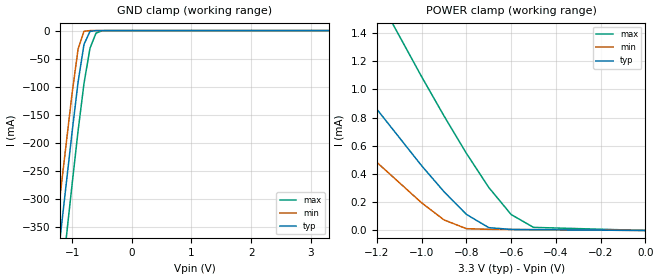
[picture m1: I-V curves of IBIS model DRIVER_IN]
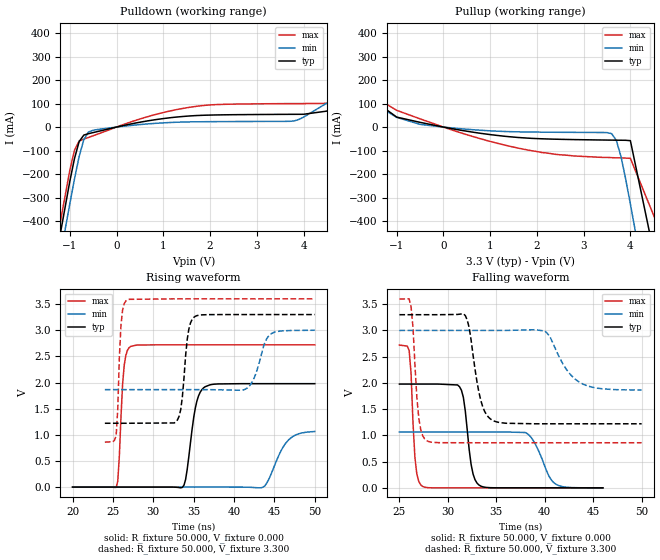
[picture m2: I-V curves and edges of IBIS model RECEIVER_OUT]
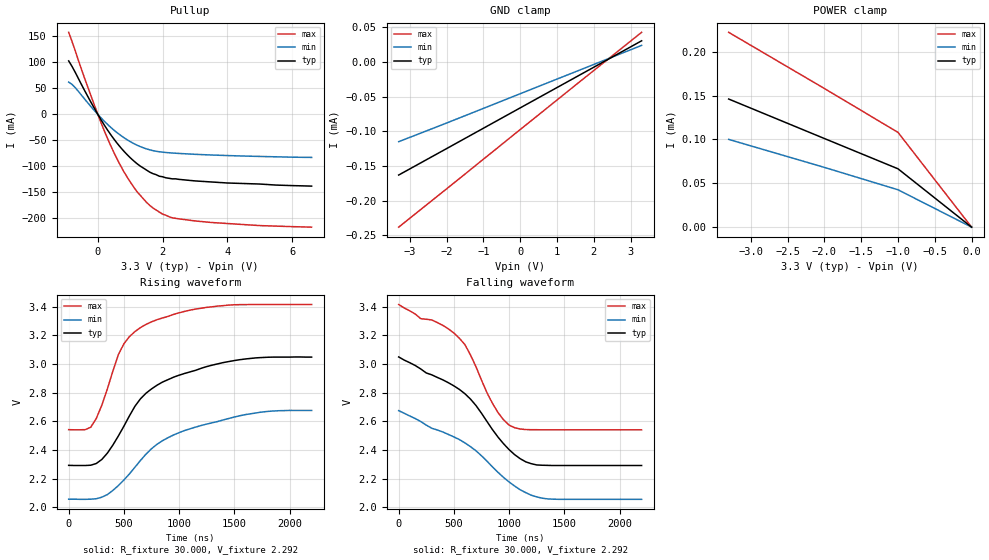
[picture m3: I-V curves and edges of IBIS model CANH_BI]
|   Texas Instruments Incorporated
|   Data Transmissions Products
|   IBIS Model for SN65HVD230
|   8D SOIC Package
[IBIS Ver]   3.2
[Comment char]   |_char
[File name]   230100.ibs
[File Rev]   3.0
[Date]   11Apr07
[Source]   File originated at Texas Instruments Incorporated.
   Data Transmission Products Group.
[Notes] Rs = 100k
[Disclaimer]
(C) Copyright Texas Instruments Incorporated 2002
   All rights reserved
  Texas Instruments Incorporated hereby grants the user of this IBIS
model a non-exclusive, nontransferable license to use this IBIS model
under the following terms.  Before using this IBIS model, the user
should read this license.  If the user does not accept these terms,
the IBIS model should be returned to Texas Instruments within 30 days.
  The user is granted this license only to use the IBIS model and
is not granted rights to sell, load, rent, lease or license the IBIS
model in whole or in part, or in modified form to anyone other than
user.  User may modify the IBIS model to suit its specific applications
but rights to derivative works and such modifications shall belong to
Texas Instruments.
  This IBIS model is provided on an "AS IS" basis and Texas Instruments
makes absolutely no warranty with respect to the information contained
herein.  TEXAS INSTRUMENTS DISCLAIMS AND CUSTOMER WAIVES ALL WARRANTIES,
EXPRESS OR IMPLIED, INCLUDING WARRANTIES OF MERCHANTABILITY OR FITNESS
FOR A PARTICULAR PURPOSE. The entire risk as to quality and performance
is with the Customer. ACCORDINGLY, IN NO EVENT SHALL THE COMPANY BE LIABLE
FOR ANY DAMAGES, WHETHER IN CONTRACT OR TORT,INCLUDING ANY LOST PROFITS
OR OTHER INCIDENTAL, CONSEQUENTIAL, EXEMPLARY, OR PUNITIVE DAMAGES ARISING
OUT OF THE USE OR APPLICATION OF THE IBIS model provided in this package.
Further, Texas Instruments reserves the right to discontinue or make changes
without notice to any product herein to improve reliability, function, or
design. Texas Instruments does not convey any license under patent rights
or any other intellectual property rights, including those of third parties.
Contact Texas Instruments at ATTN:DATA TRANSMISSIONS
[Copyright]   Copyright 2002, Texas Instruments, All Rights Reserved
[Component]   HVD230D
[Manufacturer]  Texas Instruments Incorporated
[Package]
|   typ   min   max
R_pkg   0.036   0.033   0.039
L_pkg   3.340nH   2.445nH   4.233nH
C_pkg   0.470pF   0.308pF   0.631pF
[Pin]   signal_name   model_name   R_pin   L_pin   C_pin
1   D   DRIVER_IN   0.034   4.233n   0.630p
2   GND   GND   0.038   2.445n   0.309p
3   VCC   POWER   0.039   2.448n   0.309p
4   R   RECEIVER_OUT   0.033   4.231n   0.631p
5   NC   NC
6   CANL   CANL_BI   0.039   2.450n   0.308p
7   CANH   CANH_BI   0.039   2.448n   0.309p
8   NC   NC
[Diff_pin]   inv_pin   vdiff   tdelay_typ   tdelay_min   tdelay_max
| The CANL and CANH are Diff_pins
6   7   0.500   0 0 0
| Models and submodels in the file (4): DRIVER_IN (Input), RECEIVER_OUT (Output), CANH_BI (I/O_open_source), CANL_BI (I/O_open_drain)
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|   Driver Input Model
[Model]   DRIVER_IN
Model_type   Input
|Signals   D
Vinh = 2.0
Vinl = 0.8
|   typ   min   max
C_comp   9.0pF   8.0pF   12.0pF
|   typ   min   max
[Temperature Range]   25.0   -40   85
[Voltage range]   3.3V   3.0V   3.6V
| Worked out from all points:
|   GND clamp passes 1 mA (typ) near -0.67 V on its own axis
[GND_clamp]
|   Voltage   I(typ)   I(min)   I(max)
-3.3V     -2.3A      -2.17A     -2.45A
-2V       -1.12A     -1.02A     -1.25A
-1V       -181mA     -112mA     -274mA
-900mV    -92.1mA    -33.2mA    -179mA
-800mV    -24.4mA    -1.26mA    -93.9mA
-700mV    -1.46mA    -35.1uA    -31.5mA
-600mV    -44.1uA    -25.8uA    -4.59mA
-500mV    -11.9uA    -25.7uA    -307uA
3.3V      7.64pA     -5.49uA    158pA
[Power_clamp]
| Note that the[POWER_clamp]voltage table is referenced to Vcc
| and is calculated using Vtable=Vcc - Vmeasured.
|   Voltage   I(typ)   I(min)   I(max)
-3.3V     5.22mA     3.62mA     7.96mA
-3V       4.59mA     3.17mA     7.05mA
-2.5V     3.54mA     2.42mA     5.54mA
-2V       2.5mA      1.66mA     4.03mA
-1.5V     1.46mA     913uA      2.54mA
-1V       459uA      196uA      1.09mA
-900mV    275uA      74.9uA     812uA
-800mV    114uA      12.8uA     547uA
-700mV    20.1uA     8.21uA     305uA
-600mV    7.22uA     6.92uA     113uA
-500mV    5.69uA     5.68uA     21.9uA
0V        8.14pA     7.13pA     1.06nA
|   Receiver Output MODEL
[Model]   RECEIVER_OUT
Model_type   Output
| Signals   R
Vmeas = 1.3V   |Reference voltage for timing measurements
Cref = 15pF   |Timing specification test load capacitance value
| variable   typ   min   max
C_comp   9.0pF   8.0pF   12.0pF
|   typ   min   max
[Temperature Range]   25.0   -40   85
[Voltage range]   3.3V   3.0V   3.6V
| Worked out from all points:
|   slope of the pulldown table from 0 to 0.495 V, typ, clamps not added: 24.2 ohm
|   slope of the pullup table from 0 to 0.495 V, typ, clamps not added: 28.4 ohm
|   rising waveform, R_fixture 50.000, V_fixture 0.000: 20-80 % time 1.06ns typ, 1.98ns min, 539ps max; typ from 0 V to 1.98 V
|   falling waveform, R_fixture 50.000, V_fixture 0.000: 20-80 % time 745ps typ, 1.5ns min, 417ps max; typ from 1.98 V to 0 V
|   rising waveform, R_fixture 50.000, V_fixture 3.300: 20-80 % time 735ps typ, 1.35ns min, 416ps max; typ from 1.22 V to 3.3 V
|   falling waveform, R_fixture 50.000, V_fixture 3.300: 20-80 % time 1.11ns typ, 2.21ns min, 556ps max; typ from 3.3 V to 1.22 V
[Pulldown]
|   Voltage   I(typ)   I(min)   I(max)
-3.3V     -2.74A     -2.81A     -2.71A
-2V       -1.33A     -1.42A     -1.27A
-1V       -231mA     -327mA     -184mA
-900mV    -134mA     -221mA     -98.3mA
-800mV    -61.6mA    -125mA     -59.5mA
-600mV    -28.1mA    -20.9mA    -44.1mA
1.6V      47.7mA     22.2mA     85.2mA
3.8V      54.2mA     26mA       100mA
4.5V      67.9mA     102mA      101mA
5V        150mA      166mA      113mA
6V        326mA      297mA      332mA
6.6V      434mA      363mA      469mA
[Pullup]
|   Voltage   I(typ)   I(min)   I(max)
| Note that the[Pullup]voltage table is referenced to Vcc
| and is calculated using Vtable=Vcc - Vmeasured.
-3.3V     434mA      323mA      515mA
-2.9V     362mA      284mA      446mA
-1.5V     115mA      102mA      131mA
-1V       42.4mA     41.3mA     71.2mA
-500mV    20.1mA     11.5mA     35mA
1.5V      -42.6mA    -19.9mA    -85.2mA
3.6V      -55.5mA    -28mA      -130mA
3.7V      -55.8mA    -57mA      -131mA
3.8V      -56mA      -126mA     -131mA
4V        -57.8mA    -327mA     -133mA
5V        -1.01A     -1.42A     -620mA
6.6V      -2.74A     -3.13A     -2.38A
[Ramp]
|   typ   min   max
dV/dt_r   1.25V/865ps   0.665V/1997ps   1.64V/384ps
dV/dt_f   1.25V/1107ps   0.753V/2223ps   1.63V/417ps
R_load = 50
[Rising Waveform]
R_fixture = 50.000
V_fixture = 0.000
C_fixture = 0.000
L_fixture = 0.000
|  time   V(typ)   V(min)   V(max)
20ns      50.21nV    1.391nV    38.12nV
25.4ns    50.26nV    1.391nV    -6.057mV
26.4ns    50.22nV    1.391nV    2.331V
27.2ns    50.71nV    1.343nV    2.691V
33.8ns    36.42mV    8.888nV    2.721V
35.2ns    1.508V     38.74nV    2.721V
36.4ns    1.918V     31.91nV    2.721V
43.6ns    1.978V     -647uV     2.721V
46.6ns    1.978V     876.3mV    2.721V
50ns      1.978V     1.064V     2.721V
[Falling Waveform]
R_fixture = 50.000
V_fixture = 0.000
C_fixture = 0.000
L_fixture = 0.000
|  time   V(typ)   V(min)   V(max)
25ns      1.978V     1.064V     2.721V
26ns      1.978V     1.064V     2.621V
26.6ns    1.978V     1.064V     572.7mV
27.4ns    1.978V     1.064V     26.46mV
31.2ns    1.928V     1.064V     717nV
32.6ns    262.9mV    1.064V     141nV
33.4ns    33.05mV    1.064V     101.6nV
38ns      11.46uV    1.054V     54.89nV
41ns      371.3nV    89.2mV     47.77nV
46ns      90.22nV    1.391nV    42.97nV
[Rising Waveform]
R_fixture = 50.000
V_fixture = 3.300
V_fixture_min = 3.000
V_fixture_max = 3.600
C_fixture = 0.000
L_fixture = 0.000
|  time   V(typ)   V(min)   V(max)
24ns      1.221V     1.864V     859.6mV
25.4ns    1.221V     1.864V     987.4mV
26ns      1.221V     1.864V     3.106V
26.8ns    1.221V     1.864V     3.582V
33ns      1.287V     1.864V     3.6V
34.4ns    3.018V     1.864V     3.6V
35.2ns    3.266V     1.864V     3.6V
41.4ns    3.3V       1.873V     3.6V
44.4ns    3.3V       2.907V     3.6V
50ns      3.3V       3V         3.6V
[Falling Waveform]
R_fixture = 50.000
V_fixture = 3.300
V_fixture_min = 3.000
V_fixture_max = 3.600
C_fixture = 0.000
L_fixture = 0.000
|  time   V(typ)   V(min)   V(max)
25ns      3.3V       3V         3.6V
26.2ns    3.3V       3V         3.45V
27ns      3.3V       3V         1.325V
27.8ns    3.3V       3V         901.2mV
31.8ns    3.283V     3V         859.6mV
33.4ns    1.666V     3V         859.6mV
34.6ns    1.288V     3V         859.6mV
40ns      1.221V     2.989V     859.6mV
43.6ns    1.221V     2.012V     859.6mV
50ns      1.221V     1.864V     859.6mV
[Model]   CANH_BI
Model_type   I/O_open_source
| Signals   CANH
Vinh = 0.9V
Vinl = 0.5V
Rref = 30   |Note: 60 Ohm differential load;
Vref = 2.3   |tr and tf measured single-ended
| variable   typ   min   max
C_comp   30.0pF   24.0pF   36.0pF
|   typ   min   max
[Temperature Range]   25.0   -40   85
[Voltage range]   3.3V   3.0V   3.6V
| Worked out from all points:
|   slope of the pullup table from 0 to 0.495 V, typ, clamps not added: 10.5 ohm
|   rising waveform, R_fixture 30.000, V_fixture 2.292: 20-80 % time 510ns typ, 631ns min, 324ns max; typ from 2.29 V to 3.05 V
|   falling waveform, R_fixture 30.000, V_fixture 2.292: 20-80 % time 575ns typ, 692ns min, 398ns max; typ from 3.05 V to 2.29 V
[Pullup]
|   Voltage   I(typ)   I(min)   I(max)
| Note that the[Pullup]voltage table is referenced to Vcc
| and is calculated using Vtable=Vcc - Vmeasured.
-900mV    103mA      62.2mA     158mA
-700mV    81.3mA     51.7mA     123mA
0V        30.6uA     29.3uA     34.6uA
500mV     -47.7mA    -30.4mA    -73.8mA
800mV     -70.5mA    -44.5mA    -110mA
1V        -83.3mA    -52.4mA    -130mA
1.2V      -94.3mA    -58.9mA    -148mA
1.6V      -111mA     -68.1mA    -175mA
2V        -120mA     -72.7mA    -192mA
2.5V      -125mA     -75.1mA    -201mA
5V        -134mA     -80.9mA    -214mA
6.6V      -138mA     -82.8mA    -217mA
[Power_clamp]
| Note that the[POWER_clamp]voltage table is referenced to Vcc
| and is calculated using Vtable=Vcc - Vmeasured.
|   Voltage   I(typ)   I(min)   I(max)
-3.3V     146uA      100uA      222uA
-2V       101uA      68.1uA     158uA
-1V       66.5uA     42.6uA     108uA
0V        0A         0A         0A
[GND_clamp]
|   Voltage   I(typ)   I(min)   I(max)
-3.3V     -163uA     -115uA     -238uA
-2V       -125uA     -88.2uA    -183uA
0V        -66.4uA    -46uA      -97.6uA
1.5V      -22.5uA    -14.4uA    -33.8uA
3.3V      30.2uA     23.6uA     42.4uA
[Ramp]
|   typ   min   max
dV/dt_r   0.453/510ns   0.382/625ns   0.524/323ns
dV/dt_f   0.455/573ns   0.383/695ns   0.525/398ns
R_load = 30ohm  | Note: The measurement is single-ended with 30ohm
|   to Vfixture.
[Rising Waveform]
R_fixture = 30.000
V_fixture = 2.292
V_fixture_min = 2.055
V_fixture_max = 2.541
C_fixture = 0.000
L_fixture = 0.000
|  time   V(typ)   V(min)   V(max)
0s        2.292V     2.056V     2.541V
200ns     2.293V     2.056V     2.558V
350ns     2.377V     2.088V     2.824V
450ns     2.497V     2.151V     3.064V
500ns     2.565V     2.19V      3.14V
700ns     2.795V     2.37V      3.275V
900ns     2.89V      2.485V     3.331V
1.2us     2.969V     2.57V      3.388V
1.75us    3.044V     2.664V     3.414V
2.2us     3.047V     2.675V     3.414V
[Falling Waveform]
R_fixture = 30.000
V_fixture = 2.292
V_fixture_min = 2.055
V_fixture_max = 2.541
C_fixture = 0.000
L_fixture = 0.000
|  time   V(typ)   V(min)   V(max)
0s        3.05V      2.675V     3.416V
200ns     2.966V     2.599V     3.317V
400ns     2.89V      2.526V     3.27V
550ns     2.823V     2.473V     3.18V
650ns     2.756V     2.424V     3.064V
850ns     2.542V     2.282V     2.725V
1us       2.403V     2.177V     2.574V
1.15us    2.318V     2.103V     2.543V
1.25us    2.296V     2.073V     2.542V
2.2us     2.292V     2.056V     2.541V
